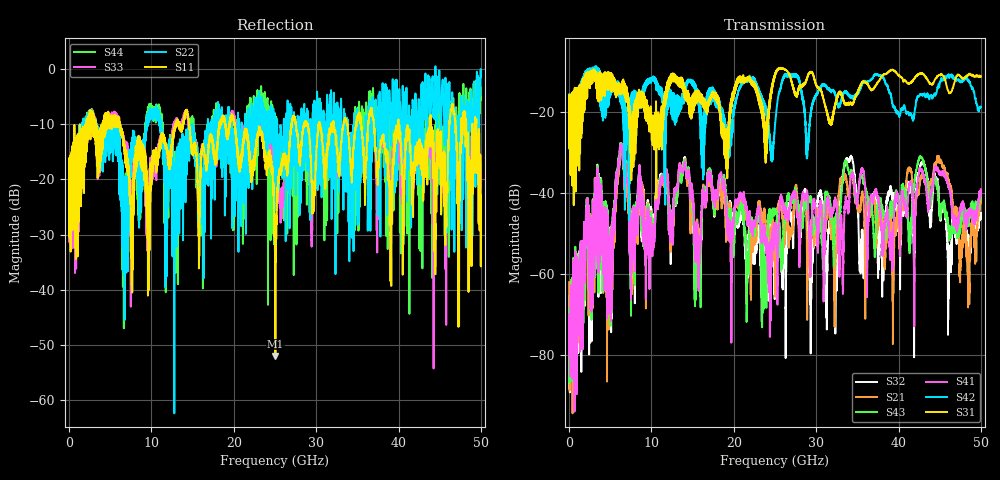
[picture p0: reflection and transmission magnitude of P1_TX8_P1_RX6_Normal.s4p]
!Keysight Technologies,N5225B,MY57041031,A.13.20.10
!Date: Friday, May 31, 2019 11:22:58
!Correction: S11(Full 4 Port(1,2,3,4))
!S12(Full 4 Port(1,2,3,4))
!S13(Full 4 Port(1,2,3,4))
!S14(Full 4 Port(1,2,3,4))
!S21(Full 4 Port(1,2,3,4))
!S22(Full 4 Port(1,2,3,4))
!S23(Full 4 Port(1,2,3,4))
!S24(Full 4 Port(1,2,3,4))
!S31(Full 4 Port(1,2,3,4))
!S32(Full 4 Port(1,2,3,4))
!S33(Full 4 Port(1,2,3,4))
!S34(Full 4 Port(1,2,3,4))
!S41(Full 4 Port(1,2,3,4))
!S42(Full 4 Port(1,2,3,4))
!S43(Full 4 Port(1,2,3,4))
!S44(Full 4 Port(1,2,3,4))
!S4P File: Measurements: <S11,S12,S13,S14>,
!<S21,S22,S23,S24>,
!<S31,S32,S33,S34>,
!<S41,S42,S43,S44>:
# Hz S  dB  R 50.0
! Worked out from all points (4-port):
!   5000 points, 10 MHz to 50 GHz, reference 50 ohm
!   strongest paths, dB at 10 MHz, 12.51 GHz, 25.01 GHz, 37.51 GHz, 50 GHz:
!     S31: -19.7, -10.8, -11.0, -12.7, -11.3
!     S42: -19.4, -15.6, -23.0, -10.9, -18.7
!     S41: -80.0, -46.5, -50.6, -41.2, -39.1
!     S43: -68.8, -45.5, -44.9, -42.8, -39.5
!     S21: -62.0, -47.7, -55.6, -46.5, -42.1
!     S32: -67.7, -47.9, -59.1, -56.7, -46.4
!   lowest |S11| = -52.0 dB at 25.05 GHz (marker M1), VSWR 1.01, Z = 49.8 - j0.14 ohm
!   |S11| at or under -10 dB: 6.192 GHz to 12.89 GHz (6.695 GHz wide, 70.2 % of centre); 20.1 GHz to 26.99 GHz (6.891 GHz wide, 29.3 % of centre); 40 GHz to 43.76 GHz (3.761 GHz wide, 8.98 % of centre)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
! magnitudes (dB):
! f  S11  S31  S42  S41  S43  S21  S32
! 10 MHz  -19.4  -19.7  -19.4  -80.0  -68.8  -62.0  -67.7
! 3.39 GHz  -13.5  -12.8  -11.6  -37.7  -36.5  -37.6  -36.5
! 5.01 GHz  -8.8  -10.5  -12.6  -68.4  -72.8  -64.9  -67.5
! 6.35 GHz  -11.8  -14.4  -15.1  -27.8  -27.7  -28.7  -28.6
! 7.76 GHz  -24.8  -31.0  -15.2  -49.5  -49.3  -51.3  -52.1
! 25.05 GHz  -52.0  -10.5  -22.2  -48.2  -44.5  -56.3  -54.3
! 50 GHz  -22.8  -11.3  -18.7  -39.1  -39.5  -42.1  -46.4
